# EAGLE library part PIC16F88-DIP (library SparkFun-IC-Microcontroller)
8-bit PIC uC RETIRED
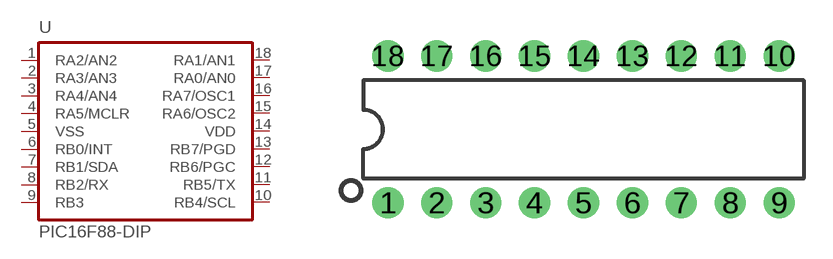
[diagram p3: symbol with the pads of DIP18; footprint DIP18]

Designator prefix -

## PIC16F88-DIP (PROD_ID: IC-08463; VALUE: PIC16F88)  [DIP18]
1  RA2/AN2
2  RA3/AN3
3  RA4/AN4
4  RA5/MCLR  in
5  VSS  pwr
6  RB0/INT
7  RB1/SDA
8  RB2/RX
9  RB3
10  RB4/SCL
11  RB5/TX
12  RB6/PGC
13  RB7/PGD
14  VDD  pwr
15  RA6/OSC2
16  RA7/OSC1
17  RA0/AN0
18  RA1/AN1

## Footprint DIP18 (pad centres in mm)
Dual In Line package type P
drill 0.813 pad 1.626: 1 -10.16,-3.81; 2 -7.62,-3.81; 3 -5.08,-3.81; 4 -2.54,-3.81; 5 0,-3.81; 6 2.54,-3.81; 7 5.08,-3.81; 8 7.62,-3.81; 9 10.16,-3.81; 10 10.16,3.81; 11 7.62,3.81; 12 5.08,3.81; 13 2.54,3.81; 14 0,3.81; 15 -2.54,3.81; 16 -5.08,3.81; 17 -7.62,3.81; 18 -10.16,3.81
